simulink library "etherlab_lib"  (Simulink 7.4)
settings: Solver=ode45  SolverMode=SingleTasking  StartTime=0.0  StopTime=10.0  RelTol=1e-3
undefined symbols (not defined in the file or in its folder): ATD4, baumer_ecatencoder, bits, Boolean, BT, CoE, CW, DC, DI8DO8, Disabled, EK1100, EK1914, ekxxxx, EL1004, EL1262, EL1904, el1xxx, EL2004, EL2262, EL2535, el2535, EL2904, el2xxx, EL3002, EL3102, EL3201, EL3204, el320x_1, EL3255, EL3314, el331x, EL3356, el3356, EL3403, el3403, EL3602, el36x2, EL3702, el37x2, EL4002, el4xxx, EL5001, el500x, EL5021, el5021, EL5101, EL5152, El5152, EL51x1, el51xx, EL6001, el60xx, EL9110, el9xxx, EP1008, ep1xxx, EP2001, ep2xxx, EP3174, EP3182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
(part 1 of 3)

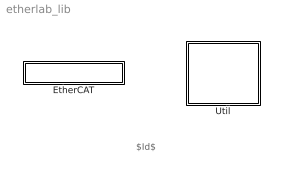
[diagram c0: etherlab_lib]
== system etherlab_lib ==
  note: $Id$
  EtherCAT : Subsystem
  Util : Subsystem

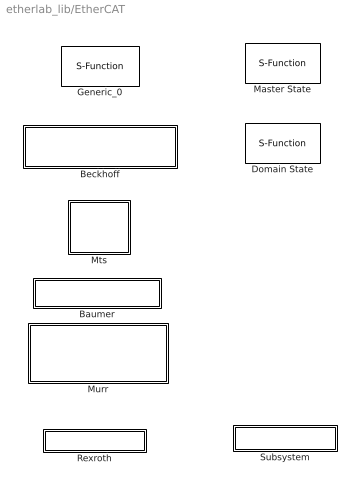
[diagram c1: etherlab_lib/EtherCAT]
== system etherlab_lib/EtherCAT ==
  Baumer : Subsystem
  Beckhoff : Subsystem
  Domain State : S-Function  FunctionName=domain_state  Parameters=master,domain,input,output,io_domain,tsample  SFunctionModules='ecrt_support'  EnableBusSupport=off  mask(Domain State){master=0, domain=0, direction=Input and Output, io_domain=on, tsample=0}
      mask prompts: io_domain "Tx and RxPdo in one domain"; tsample "Sample Time"
      mask help: Displays the following domain state information: * Working Counter * Domain state: 0 - No slaves 1 - Domain incomplete 2 - Domain complete
      mask init:
      | switch direction
      |     case 1
      |         input = 1;
      |         output = 0;
      |     case 2
      |         input = 0;
      |         output = 1;
      |     case 3
      |         input = 1;
      |         output = 1;
      | end
  Generic_0 : S-Function  FunctionName=ec_slave3  Parameters=Address,rv.SlaveConfig,rv.PortConfig,debug,tsample,param  SFunctionModules='ecrt_support'  EnableBusSupport=off  mask(Generic EtherCAT Slave){master=0, index=1, rv=[], param=[], tsample=0, debug=0}
      mask prompts: index "Slave Index"; rv "EtherCAT Slave Configuration struct. (SlaveConfig, PortConfig)"; param "Block Parameters"; tsample "Sample Time"
      mask help: The generic EtherCAT Slave is used to create any slave not contained in this library. A mask input variable, <b>EtherCAT Slave Configuration</b>, has to be set up by the user. This configures the slave.
      mask init:
      | Address = EtherCATSlave.formatAddress(master,index,tsample);
      | 
      | inputnames = {};
      | outputnames = {};
      | 
      | if ~isfield(rv,'PortConfig') || isempty(rv)
      |    rv.PortConfig = [];
      | else
      |     rv.PortConfig.swap_io = EtherCATSlave.shouldSwapIoPorts();
      |     if isfield(rv.PortConfig, 'output')
      |         if isfield(rv.PortConfig.output, 'portname')
      |             outputnames = {rv.PortConfig.output.portname};
      |         end
      |     end
      |     if isfield(rv.PortConfig, 'input')
      |         if isfield(rv.PortConfig.input, 'portname')
      |             inputnames = {rv.PortConfig.input.portname};
      |         end
      |     end
      | end
      | 
      | 
      | if ~isfield(rv,'SlaveConfig') || isempty(rv)
      |    rv.SlaveConfig = [];
      | end
      | 
      | if ~isfield(rv.SlaveConfig,'description') || isempty(rv)
      |    slave_name = 'unknown';
      | else
      |    slave_name = rv.SlaveConfig.description;
      | end
      | 
      | if isempty(inputnames) && isempty(outputnames)
      |     EtherCATSlave.setPortNames({}, {}, ...
      |         sprintf('GenericSlave\\n%s\\nM:%i Idx:%s',...
      |             slave_name,master,mat2str(index)))
      | else
      |     EtherCATSlave.setPortNames(inputnames,...
      |             outputnames)
      | end
      | 
      | set_param(gcb,'AttributesFormatString',...
      |         sprintf('GenericSlave\n%s\nM:%i Idx:%s',...
      |         slave_name,master,mat2str(index)))
  Master State : S-Function  FunctionName=master_state  Parameters=master,devices,reset,sync_dec,tsample,scan_progess  SFunctionModules='ecrt_support'  EnableBusSupport=off  mask(Master State){master=0, devices=1, reset=off, sync_dec=0, tsample=0, scan_progess=off}
      mask prompts: devices "Device Count"; reset "Reset Port"; sync_dec "Reference Clock Sync Decimation"; tsample "Sample Time"; scan_progess "Scan Progress Port"
      mask help: Outputs master state: * number of responding slaves * Slave states * Link up * Scan Progress (optional) Enabling <b>Master Reset</b> forces the master to reset the bus and scan for new slaves Enabling <b>Scan Progress</b> will add a forth Output Port. This requires EtherCAT &gt; 1.6.0. The first element is the scan index, the second element the total number of slaves. If both numbers are equal, the network scan has finished.
  Mts : Subsystem
  Murr : Subsystem
  Rexroth : Subsystem
  Subsystem : Subsystem

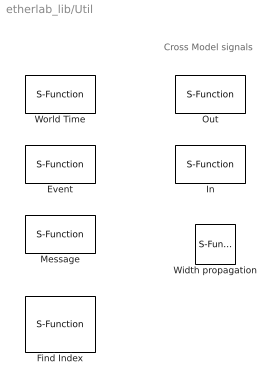
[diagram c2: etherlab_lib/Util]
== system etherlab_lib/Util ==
  note: Cross Model signals
  Event : S-Function  FunctionName=event  Parameters=width,singleshot,dtype,tsample  EnableBusSupport=off  mask(Trigger Events){width=-1, singleshot=on, dtype_str=Boolean, tsample=eval(get_param(bdroot,'FixedStep'))}
      mask prompts: singleshot "Single shot"; dtype_str "Data Type"; tsample "Sample Time"
      mask help: This block is used to generate an events on its output. Checking the "One Shot" option will generate only one event, otherwise a whole chain of events is generated for every count that the parameter value was incremented. Width specifies output port width. If -1 is chosen, an input port appears, propagating the width to the output.
      mask init:
      | switch dtype_str
      |     case 'Unsigned Integer'
      |         dtype = 32;
      |     case 'Boolean'
      |         dtype = 1;
      |     case 'Dynamically Typed';
      |         dtype = -1;
      |     otherwise
      |         dtype = 1;
      | end
  Find Index : S-Function  FunctionName=findidx  Parameters=cmp,tsample  EnableBusSupport=off  mask(Find MinMax){cmp=First Minimum, tsample=-1}
      mask prompts: cmp "Comparison"; tsample "Sample Time"
      mask help: This block takes a vector input and outputs: 1: Found count 2: Found Index (zero based) 3: Value
  In : S-Function  FunctionName=rtipc_rx  Parameters=varname,dtype,len,force,tsample  SFunctionModules='rtipc'  EnableBusSupport=off  mask(Generic Output Port){varname='SIG01', dtype=double, len=1, force=off, tsample=0}
      mask prompts: varname "Signal Name"; dtype "Data Type"; len "Vector Length"; force "Enable value forcing"; tsample "Sample Time (-1 for inherited)"
      mask help: RealTime Interprocess Communication input Signal Name: Name of signal to connect to (string) Data Type: Signal's data type Vector Length: Number of elements Enable Force Value: Adds additional parameters to force the output value
  Message : S-Function  FunctionName=etl_message  Parameters=prio,message_text,reset,invert,confirm,tsample  EnableBusSupport=off  mask(Generate system message){prio=Error, message_text={}, reset=on, invert=off, confirm=[], tsample=-1}
      mask prompts: prio "Priority"; message_text "Message List"; reset "External Reset"; invert "Invert Input"; confirm "Input confirm delay [s]"; tsample "Sample Time (-1 for inherited)"
      mask help: This block generates a system message when the input port 1 is true. The current time is output on output port.
      mask init:
      | m = {'Emergency', 'Alert', 'Critical', 'Error', ...
      |     'Warning', 'Notice', 'Information', 'Debug'};
      | cmap = [
      |     1 0 1;
      |     1 0 1;
      |     1 0 1;
      |     1 0 0;
      |     1 0.5 0.0;
      |     0 0 1;
      |     0 0 1;
      |     0 0 1;
      |     ]; 
      | c = cmap(prio,:);
      | priority = m{prio};
  Out : S-Function  FunctionName=rtipc_tx  Parameters=varname,force,tsample  SFunctionModules='rtipc'  EnableBusSupport=off  mask(Generic Output Port){varname='SIG01', force=off, tsample=-1}
      mask prompts: varname "Signal Name"; force "Enable value forcing"; tsample "Sample Time (-1 for inherited)"
  Width propagation : S-Function  FunctionName=propagate_width  Parameters=count,width  EnableBusSupport=off  mask(Propagate width){count=2, width=-1}
      mask prompts: count "Port Count"; width "Width (-1 = inherited)"
      mask help: This block forces all input ports to have the same width if width is a positive integer, otherwise the width of port 1 is propagated to all ports.
      mask init:
      | if width <= 0
      |     width = -1;
      |     widthstr = '=';
      | else
      |     widthstr = num2str(width);
      | end
  World Time : S-Function  FunctionName=world_time  Parameters=tsample  EnableBusSupport=off  mask(World Time){tsample=0}
      mask prompts: tsample "Sample Time"
      mask help: Outputs the current world time for the given sample time.

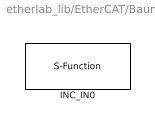
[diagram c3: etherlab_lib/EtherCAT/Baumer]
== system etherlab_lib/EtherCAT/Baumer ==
  INC_IN0 : S-Function  LoadFcn=baumer_ecatencoder().checkModelName  FunctionName=ec_slave3  Parameters=Address,rv.SlaveConfig,rv.PortConfig,debug,tsample  SFunctionModules='ecrt_support'  EnableBusSupport=off  mask(Baumer && Thalheim ATD Encoder){master=0, index=1, model=BT ATD4, revision=[1 2], direction=CW, tsample=0, debug=, dc_mode=Free Run/SM-Synchron, dc_assign_activate=, dc_cycle0=[], dc_cycle0_factor=[], dc_shift0=[], dc_shift0_factor=[], dc_shift0_input=off, dc_cycle1=[], dc_cycle1_factor=[], dc_shift1=[], dc_shift1_factor=[]}
      mask prompts: index "Slave Index"; model "Device Model"; direction "Counting direction"; tsample "Sample Time (-1 for inherited)"; dc_mode "Mode"; dc_assign_activate "Assign Activate"; dc_cycle0 "Cycle Time Sync 0"; dc_cycle0_factor "Factor"; dc_shift0 "Shift Time Sync0"; dc_shift0_factor "Factor"; dc_shift0_input "Shift Time0 Input"; dc_cycle1 "Cycle Time Sync1"; dc_cycle1_factor "Factor"; dc_shift1 "Shift Time Sync1"; dc_shift1_factor "Factor"
      mask help: Baumer & Thalheim ATD Encoder
      mask init:
      | Address = EtherCATSlave.formatAddress(master,index,tsample);
      | 
      | rv = baumer_ecatencoder(model).configure(direction-1,...
      |     [dc_mode, dc_assign_activate, ...
      |      dc_cycle0, dc_cycle0_factor, ...
      |      dc_shift0, dc_shift0_factor, dc_shift0_input, ...
      |      dc_cycle1, dc_cycle1_factor, ...
      |      dc_shift1, dc_shift1_factor]);
      | 
      | rv.PortConfig.swap_io = EtherCATSlave.shouldSwapIoPorts();
